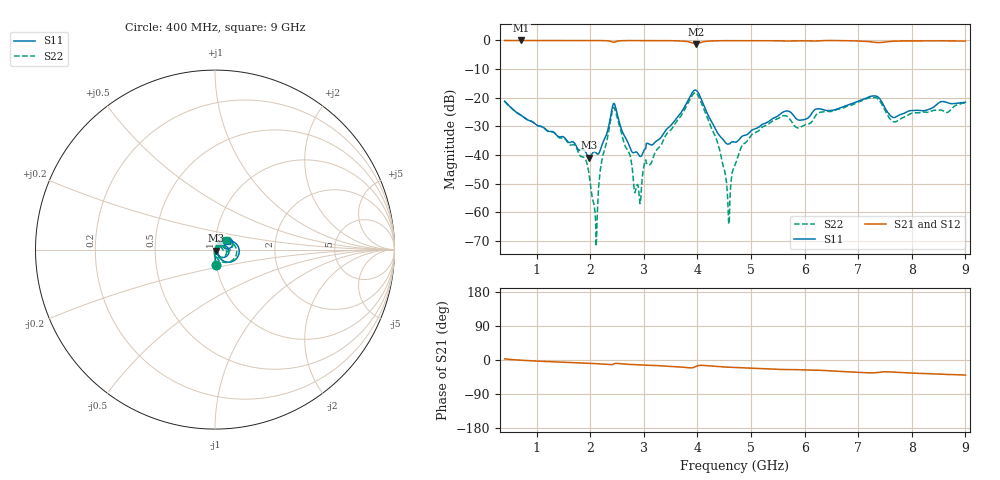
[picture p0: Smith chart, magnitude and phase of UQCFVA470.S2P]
!  Part Number  UQCFVA470  Mounting Orientation: Horizontal
!  Description: Ultra Low ESR Microwave capacitors
!  Application: Coupling, Bypass, Tuning, DC Block
!  Filters, Matching
# GHZ S DB R 50
! Freq  |S11|  S11 Ph  |S21|  S21 Ph  |S12|  S12 Ph  |S22|  S22 Ph
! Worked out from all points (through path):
!   801 points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, 400 MHz to 9 GHz, reference 50 ohm
!   highest |S21| = -0.02 dB at 712 MHz (marker M1); lowest = -1.2 dB at 3.969 GHz (marker M2)
!   group delay of S21, straight-line fit = 12.6 ps
!   lowest |S11| = -41.0 dB at 1.98 GHz (marker M3), VSWR 1.02, Z = 50.7 - j0.533 ohm
!   |S11| at or under -10 dB: start of sweep to end of sweep
!   |S22| runs from -71.9 to -18.2 dB; largest |S21 - S12| = 0.007
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0.4  -21.26 -86.6  -0.04 3.0  -0.04 3.0  -21.24 -86.7
0.712  -26.23 -88.8  -0.02 -0.6  -0.03 -0.6  -26.19 -90.3
1.841  -38.22 -57.2  -0.03 -7.9  -0.03 -8.0  -40.65 -113.5
1.98  -40.98 -36.0  -0.05 -8.8  -0.04 -8.9  -47.34 -102.6
2.077  -38.87 -17.9  -0.06 -9.4  -0.06 -9.5  -58.30 -149.2
2.109  -39.34 -13.4  -0.06 -9.6  -0.06 -9.7  -71.89 -110.5
2.206  -37.19 17.8  -0.08 -10.3  -0.08 -10.4  -42.89 55.7
2.432  -22.10 -5.1  -0.67 -11.0  -0.67 -11.1  -23.43 -12.5
2.754  -38.11 -46.2  -0.06 -11.7  -0.06 -11.8  -41.31 -108.1
2.894  -39.72 -9.4  -0.07 -12.7  -0.07 -12.9  -51.02 154.6
3.023  -37.92 25.2  -0.08 -13.5  -0.08 -13.6  -42.20 61.7
3.27  -34.69 29.9  -0.07 -15.0  -0.07 -15.1  -37.61 78.0
3.969  -17.38 -11.8  -1.22 -17.2  -1.22 -17.4  -18.27 -16.5
4.378  -32.44 -49.9  -0.13 -17.4  -0.13 -17.6  -35.91 -90.9
4.571  -36.24 -12.7  -0.09 -18.9  -0.09 -19.1  -58.42 -79.2
4.7  -35.55 12.1  -0.08 -19.8  -0.08 -20.0  -43.53 85.8
4.861  -33.27 30.9  -0.08 -20.8  -0.08 -21.0  -36.11 73.8
5.42  -27.14 50.7  -0.11 -24.1  -0.11 -24.3  -27.97 56.2
6.141  -25.29 60.2  -0.21 -27.1  -0.21 -27.3  -28.28 64.6
7.269  -19.41 31.3  -0.57 -34.0  -0.57 -34.3  -19.95 20.6
7.57  -25.62 10.3  -0.41 -31.2  -0.41 -31.5  -26.85 -2.9
9  -21.61 36.5  -0.24 -39.6  -0.24 -40.0  -21.89 39.5
